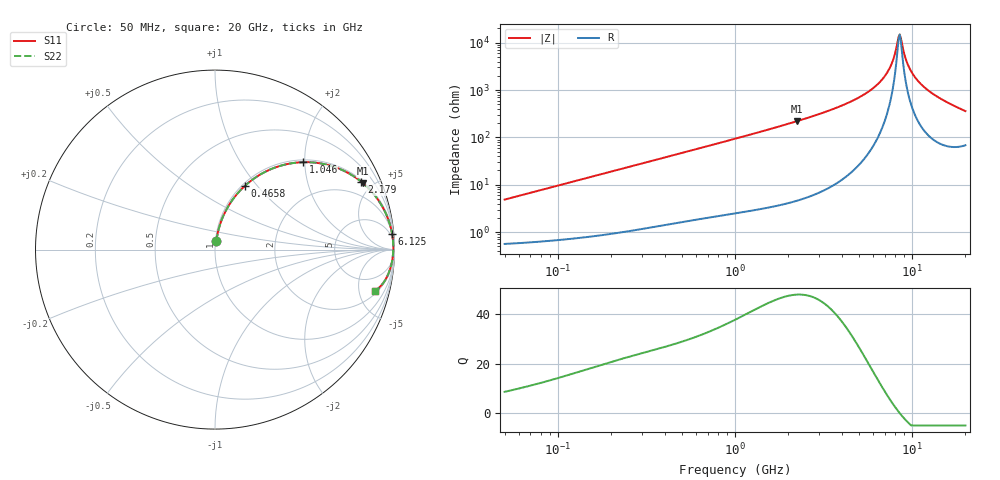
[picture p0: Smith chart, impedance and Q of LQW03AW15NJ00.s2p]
!Murata Part Number: LQW03AW15NJ00
!These Parameters are Measured in Series Mode Connection
!  o--[Z]--o
!Port1  Port2
!  o-------o
!Freq. Start=50[MHz] Stop=20[GHz], 401[Steps]
# Hz S RI R 50
!Freq.(Hz) S11(Real) S11(Imag) S21(Real) S21(Imag) S12(Real) S12(Imag) S22(Real) S22(Imag)
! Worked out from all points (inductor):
!   401 points, 50 MHz to 20 GHz, reference 50 ohm
!   read as one part in series: L = 15.3 nH near 51.52 MHz
!   highest Q = 47.8 at 2.245 GHz (marker M1), where L = 15.6 nH
!   self-resonance near 8.389 GHz
!   S11 on the Smith chart (normalised r, x): 50 MHz: 1.01, +0.10; 465.8 MHz: 1.03, +0.87; 1.046 GHz: 1.05, +1.96; 2.179 GHz: 1.09, +4.26; 6.125 GHz: 2, +23; 20 GHz: 2.36, -7.05
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5e7  0.00788 0.0476  0.9921 -0.0476  0.9921 -0.0476  0.00788 0.0476
1.364002e8  0.0238 0.126  0.9762 -0.126  0.9762 -0.126  0.0238 0.126
3.721004e8  0.1181 0.3041  0.8819 -0.3041  0.8819 -0.3041  0.1181 0.3041
4.658406e8  0.1686 0.3571  0.8314 -0.3571  0.8314 -0.3571  0.1686 0.3571
1e9  0.4672 0.4858  0.5328 -0.4858  0.5328 -0.4858  0.4672 0.4858
1.045961e9  0.4894 0.487  0.5106 -0.487  0.5106 -0.487  0.4894 0.487
2.179053e9  0.8147 0.3782  0.1853 -0.3782  0.1853 -0.3782  0.8147 0.3782
2.245319e9  0.8245 0.3701  0.1755 -0.3701  0.1755 -0.3701  0.8245 0.3701
2.728004e9  0.88 0.3145  0.12 -0.3145  0.12 -0.3145  0.88 0.3145
4.472136e9  0.9643 0.1706  0.0357 -0.1706  0.0357 -0.1706  0.9643 0.1706
6.125241e9  0.9872 0.0852  0.0128 -0.0852  0.0128 -0.0852  0.9872 0.0852
6.802353e9  0.991 0.0578  0.00904 -0.0578  0.00904 -0.0578  0.991 0.0578
7.442007e9  0.9928 0.0345  0.00717 -0.0345  0.00717 -0.0345  0.9928 0.0345
7.901521e9  0.9934 0.019  0.0066 -0.019  0.0066 -0.019  0.9934 0.019
8.264682e9  0.9935 0.00745  0.00653 -0.00745  0.00653 -0.00745  0.9935 0.00745
8.516016e9  0.9933 -0.000286  0.00666 0.000286  0.00666 0.000286  0.9933 -0.000286
8.644534e9  0.9932 -0.00415  0.00678 0.00415  0.00678 0.00415  0.9932 -0.00415
9.178299e9  0.9924 -0.0197  0.0076 0.0197  0.0076 0.0197  0.9924 -0.0197
9.600142e9  0.9914 -0.0314  0.00861 0.0314  0.00861 0.0314  0.9914 -0.0314
1.098561e10  0.9862 -0.0669  0.0138 0.0669  0.0138 0.0669  0.9862 -0.0669
1.396067e10  0.9668 -0.1326  0.0332 0.1326  0.0332 0.1326  0.9668 -0.1326
2e10  0.8897 -0.2311  0.1103 0.2311  0.1103 0.2311  0.8897 -0.2311
